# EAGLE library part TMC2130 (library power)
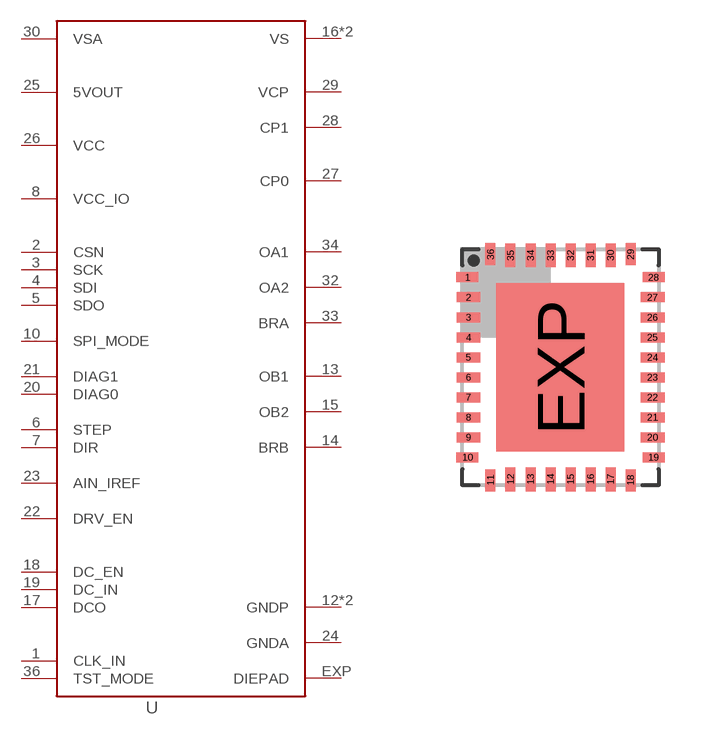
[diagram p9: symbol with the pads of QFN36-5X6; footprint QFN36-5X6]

Designator prefix U

## TMC2130  [QFN36-5X6]
1  CLK_IN
2  CSN
3  SCK
4  SDI
5  SDO
6  STEP
7  DIR
8  VCC_IO
10  SPI_MODE
12  GNDP
13  OB1
14  BRB
15  OB2
16  VS
17  DCO
18  DC_EN
19  DC_IN
20  DIAG0
21  DIAG1
22  DRV_EN
23  AIN_IREF
24  GNDA
25  5VOUT
26  VCC
27  CP0
28  CP1
29  VCP
30  VSA
31  VS
32  OA2
33  BRA
34  OA1
35  GNDP
36  TST_MODE
EXP  DIEPAD

## Footprint QFN36-5X6 (pad centres in mm)
QFN 32 5 x 5 mm Source: http://datasheets.maxim-ic.com/en/ds/MAX7042.pdf
smd 0.55 x 0.25: 1 -2.325,1.75; 10 -2.325,-2.75; 19 2.325,-2.75; 28 2.325,1.75
smd 0.6 x 0.25: 2 -2.3,1.25; 3 -2.3,0.75; 4 -2.3,0.25; 5 -2.3,-0.25; 6 -2.3,-0.75; 7 -2.3,-1.25; 8 -2.3,-1.75; 9 -2.3,-2.25; 20 2.3,-2.25; 21 2.3,-1.75; 22 2.3,-1.25; 23 2.3,-0.75; 24 2.3,-0.25; 25 2.3,0.25; 26 2.3,0.75; 27 2.3,1.25
smd 0.25 x 0.55: 11 -1.75,-3.325; 18 1.75,-3.325; 29 1.75,2.325; 36 -1.75,2.325
smd 0.25 x 0.6: 12 -1.25,-3.3; 13 -0.75,-3.3; 14 -0.25,-3.3; 15 0.25,-3.3; 16 0.75,-3.3; 17 1.25,-3.3; 30 1.25,2.3; 31 0.75,2.3; 32 0.25,2.3; 33 -0.25,2.3; 34 -0.75,2.3; 35 -1.25,2.3
smd 3.2 x 4.2: EXP 0,-0.5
